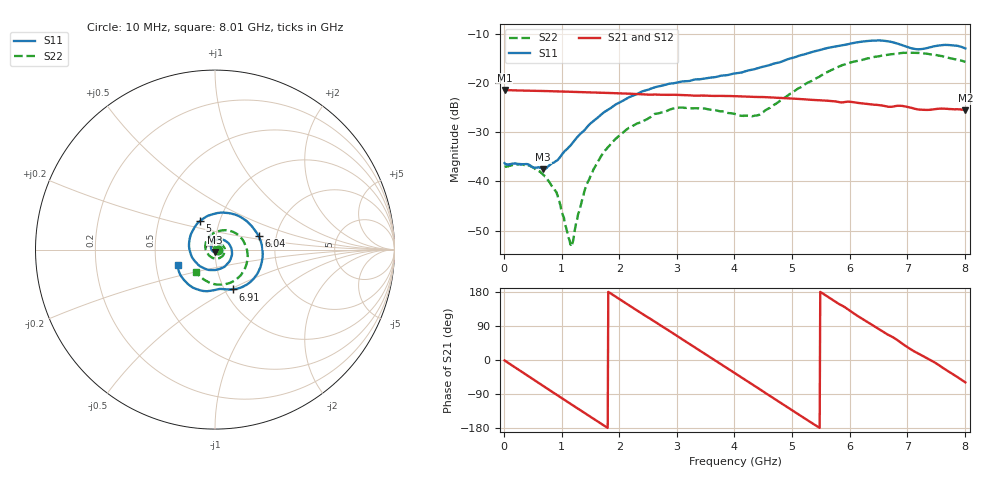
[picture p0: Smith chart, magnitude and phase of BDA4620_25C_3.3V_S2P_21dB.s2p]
!Agilent Technologies,E5071B,MY42404982,A.09.10
!Date: Wed May 06 08:53:17 2026
!Data & Calibration Information:
!Freq	S11:SOLT2(ON)	S21:SOLT2(ON)	S12:SOLT2(ON)	S22:SOLT2(ON)
# Hz S RI R 50
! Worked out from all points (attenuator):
!   801 points, 10 MHz to 8.01 GHz, reference 50 ohm
!   highest |S21| = -21.41 dB at 10 MHz (marker M1); lowest = -25.5 dB at 8.01 GHz (marker M2)
!   lowest |S11| = -37.5 dB at 680 MHz (marker M3), VSWR 1.03, Z = 49.7 - j1.29 ohm
!   |S11| at or under -10 dB: start of sweep to end of sweep
!   |S22| runs from -53.2 to -13.8 dB; largest |S21 - S12| = 0.00035
!   S11 on the Smith chart (normalised r, x): 10 MHz: 1.03, -0.00; 5 GHz: 0.81, +0.27; 6.04 GHz: 1.61, +0.26; 6.91 GHz: 1.09, -0.52; 8.01 GHz: 0.65, -0.12
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1e7  0.0153 -0.00106  0.085 -0.00177  0.0852 -0.00179  0.014 -0.000482
4.2e8  0.0086 -0.0121  0.0618 -0.0566  0.0618 -0.0567  0.0136 -0.00507
6.8e8  -0.00276 -0.013  0.0306 -0.0773  0.0305 -0.0775  0.00925 -0.00713
9.2e8  -0.0148 -0.00688  -0.00338 -0.0823  -0.00344 -0.0824  0.00352 -0.00656
1.16e9  -0.0222 0.00776  -0.0361 -0.0733  -0.0361 -0.0734  -0.00191 -0.00122
1.2e9  -0.0227 0.0107  -0.0409 -0.0705  -0.041 -0.0706  -0.0025 4.59e-05
1.35e9  -0.0222 0.0223  -0.0573 -0.0573  -0.0573 -0.0574  -0.00408 0.00478
1.53e9  -0.0159 0.0369  -0.0714 -0.0369  -0.0715 -0.0369  -0.00386 0.0117
1.77e9  0.00199 0.052  -0.0794 -0.00513  -0.0795 -0.0051  0.000542 0.0211
2.15e9  0.0448 0.0547  -0.0651 0.0434  -0.0652 0.0436  0.0174 0.0299
2.68e9  0.0926 0.00268  -0.00671 0.0761  -0.00663 0.0762  0.0452 0.0196
3.08e9  0.0824 -0.0629  0.0423 0.0628  0.0425 0.0628  0.056 -0.00796
4.01e9  -0.0889 -0.0885  0.0603 -0.0422  0.0604 -0.0423  -0.0114 -0.0473
4.42e9  -0.1428 0.00319  0.0185 -0.0699  0.0184 -0.0699  -0.0458 -0.0127
5e9  -0.083 0.1593  -0.0471 -0.0514  -0.0472 -0.0514  -0.032 0.0734
5.35e9  0.0276 0.2057  -0.0658 -0.0155  -0.0659 -0.0155  0.0232 0.1035
6.04e9  0.2424 0.0764  -0.0379 0.0519  -0.038 0.052  0.1541 0.0545
6.37e9  0.2616 -0.0659  -0.00465 0.0605  -0.00457 0.0606  0.1805 -0.0165
6.68e9  0.1877 -0.188  0.0238 0.0523  0.0238 0.0525  0.1715 -0.0919
6.91e9  0.1001 -0.2221  0.0426 0.0404  0.0427 0.0405  0.1433 -0.1434
7.57e9  -0.0904 -0.2247  0.0531 -0.0149  0.0532 -0.0148  -0.0179 -0.1884
8.01e9  -0.2084 -0.0853  0.0273 -0.0456  0.0275 -0.0457  -0.1041 -0.127
